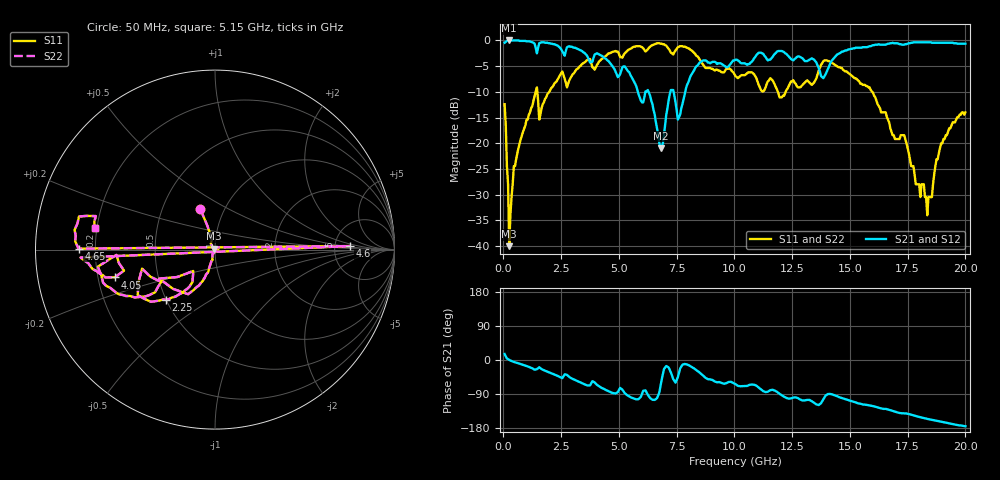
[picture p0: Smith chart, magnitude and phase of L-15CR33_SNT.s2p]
#	mhz	s	ma	r	50
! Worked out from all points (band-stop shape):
!   400 points, 50 MHz to 20 GHz, reference 50 ohm
!   highest |S21| = 0.00 dB at 250 MHz (marker M1); lowest = -20.9 dB at 6.8 GHz (marker M2)
!   |S21| within 3 dB of the highest: start of sweep to 3.62 GHz; 14.39 GHz to end of sweep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
!   lowest |S11| = -40.0 dB at 250 MHz (marker M3), VSWR 1.02, Z = 49.2 + j0.569 ohm
!   |S11| at or under -10 dB: start of sweep to 1.394 GHz; 1.467 GHz to 1.981 GHz (514.3 MHz wide, 29.8 % of centre); 15.97 GHz to end of sweep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
!   |S22| runs from -40.0 to -0.5 dB; largest |S21 - S12| = 0
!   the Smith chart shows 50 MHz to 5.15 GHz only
!   S11 on the Smith chart (normalised r, x): 50 MHz: 0.77, +0.37; 2.25 GHz: 0.50, -0.33; 4.05 GHz: 0.27, -0.13; 4.6 GHz: 6.94, +0.62; 4.65 GHz: 0.14, +0.00; 5.15 GHz: 0.19, +0.09
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50  0.24 110.0  0.95 15.6  0.95 15.6  0.24 110.0
250  0.01 144.7  1 0.2  1 0.2  0.01 144.7
450  0.06 -103.3  1 -5.1  1 -5.1  0.06 -103.3
750  0.11 -107.6  0.99 -10.9  0.99 -10.9  0.11 -107.6
2250  0.39 -134.4  0.91 -39.2  0.91 -39.2  0.39 -134.4
3400  0.59 -155.0  0.79 -60.9  0.79 -60.9  0.59 -155.0
4050  0.58 -164.5  0.75 -65.6  0.75 -65.6  0.58 -164.5
4550  0.75 -176.6  0.63 -82.4  0.63 -82.4  0.75 -176.6
4600  0.75 1.5  0.61 -83.9  0.61 -83.9  0.75 1.5
4650  0.76 179.6  0.59 -85.5  0.59 -85.5  0.76 179.6
5150  0.68 169.8  0.55 -78.5  0.55 -78.5  0.68 169.8
6700  0.94 137.3  0.12 -93.1  0.12 -93.1  0.94 137.3
6800  0.93 133.4  0.09 -68.8  0.09 -68.8  0.93 133.4
7250  0.76 117.6  0.33 -32.9  0.33 -32.9  0.76 117.6
7550  0.86 118.4  0.17 -45.7  0.17 -45.7  0.86 118.4
8550  0.63 69.9  0.62 -36.1  0.62 -36.1  0.63 69.9
10050  0.45 72.8  0.65 -63.9  0.65 -63.9  0.45 72.8
13350  0.37 70.0  0.67 -108.8  0.67 -108.8  0.37 70.0
14250  0.6 16.2  0.65 -91.2  0.65 -91.2  0.6 16.2
16700  0.16 9.8  0.93 -131.5  0.93 -131.5  0.16 9.8
18350  0.02 87.3  0.96 -155.5  0.96 -155.5  0.02 87.3
20000  0.2 -59.7  0.93 -174.8  0.93 -174.8  0.2 -59.7
